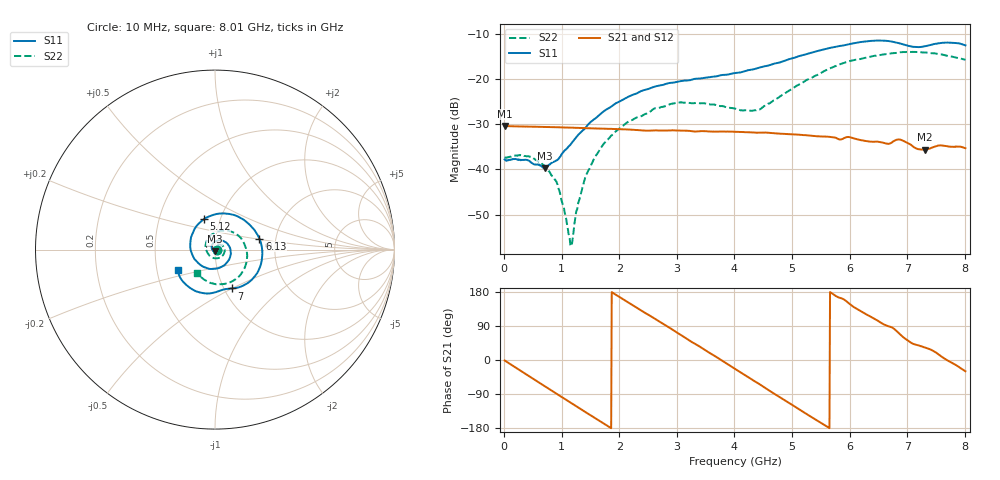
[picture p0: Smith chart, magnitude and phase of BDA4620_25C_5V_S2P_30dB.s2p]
!Agilent Technologies,E5071B,MY42404982,A.09.10
!Date: Wed May 06 09:05:00 2026
!Data & Calibration Information:
!Freq	S11:SOLT2(ON)	S21:SOLT2(ON)	S12:SOLT2(ON)	S22:SOLT2(ON)
# Hz S RI R 50
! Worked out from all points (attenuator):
!   801 points, 10 MHz to 8.01 GHz, reference 50 ohm
!   highest |S21| = -30.37 dB at 10 MHz (marker M1); lowest = -35.6 dB at 7.31 GHz (marker M2)
!   lowest |S11| = -39.6 dB at 710 MHz (marker M3), VSWR 1.02, Z = 49.7 - j1 ohm
!   |S11| at or under -10 dB: start of sweep to end of sweep
!   |S22| runs from -57.0 to -13.9 dB; largest |S21 - S12| = 0.00018
!   S11 on the Smith chart (normalised r, x): 10 MHz: 1.03, -0.00; 5.12 GHz: 0.84, +0.29; 6.13 GHz: 1.64, +0.22; 7 GHz: 1.09, -0.50; 8.01 GHz: 0.64, -0.15
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1e7  0.0129 -0.000777  0.0303 -0.000612  0.0303 -0.000666  0.0135 -0.000459
4.4e8  0.00762 -0.00983  0.0218 -0.0204  0.0218 -0.0205  0.0131 -0.00473
7.1e8  -0.00269 -0.0101  0.0104 -0.0278  0.0104 -0.0278  0.00856 -0.00666
9.3e8  -0.0117 -0.005  -0.000348 -0.0294  -0.000422 -0.0294  0.00358 -0.00575
1.16e9  -0.0179 0.00667  -0.0113 -0.0268  -0.0114 -0.0268  -0.00121 -0.000722
1.19e9  -0.0184 0.00855  -0.0127 -0.0261  -0.0127 -0.0262  -0.00166 0.000135
1.35e9  -0.0184 0.019  -0.019 -0.0217  -0.0191 -0.0217  -0.00321 0.00488
1.53e9  -0.0136 0.0319  -0.0244 -0.015  -0.0244 -0.015  -0.00293 0.0114
1.77e9  0.00114 0.0458  -0.028 -0.00429  -0.028 -0.00427  0.00112 0.0204
2.15e9  0.0387 0.0505  -0.0246 0.0129  -0.0246 0.013  0.0173 0.0289
2.68e9  0.0847 0.00742  -0.00611 0.0263  -0.00608 0.0264  0.0441 0.0192
3.06e9  0.0814 -0.0494  0.0106 0.0248  0.0106 0.0248  0.055 -0.00588
4.01e9  -0.0748 -0.0901  0.024 -0.0104  0.0241 -0.0104  -0.0106 -0.0462
4.43e9  -0.1342 -0.00729  0.0115 -0.0229  0.0115 -0.0229  -0.0448 -0.0113
5.12e9  -0.0623 0.1694  -0.0155 -0.0187  -0.0156 -0.0187  -0.0152 0.0862
5.35e9  0.00904 0.1984  -0.0208 -0.0112  -0.0208 -0.0113  0.0234 0.1018
6.13e9  0.2472 0.0618  -0.0151 0.0155  -0.0151 0.0155  0.162 0.0353
6.68e9  0.2041 -0.1687  0.000404 0.0192  0.000386 0.0193  0.1698 -0.0898
7e9  0.095 -0.2164  0.012 0.0157  0.0121 0.0157  0.1242 -0.1575
7.31e9  0.0224 -0.2314  0.0139 0.00899  0.014 0.00906  0.0511 -0.1916
7.65e9  -0.1045 -0.2328  0.0183 0.00109  0.0182 0.00105  -0.0322 -0.1822
8.01e9  -0.2089 -0.1137  0.0149 -0.00851  0.0149 -0.00853  -0.1026 -0.1283
